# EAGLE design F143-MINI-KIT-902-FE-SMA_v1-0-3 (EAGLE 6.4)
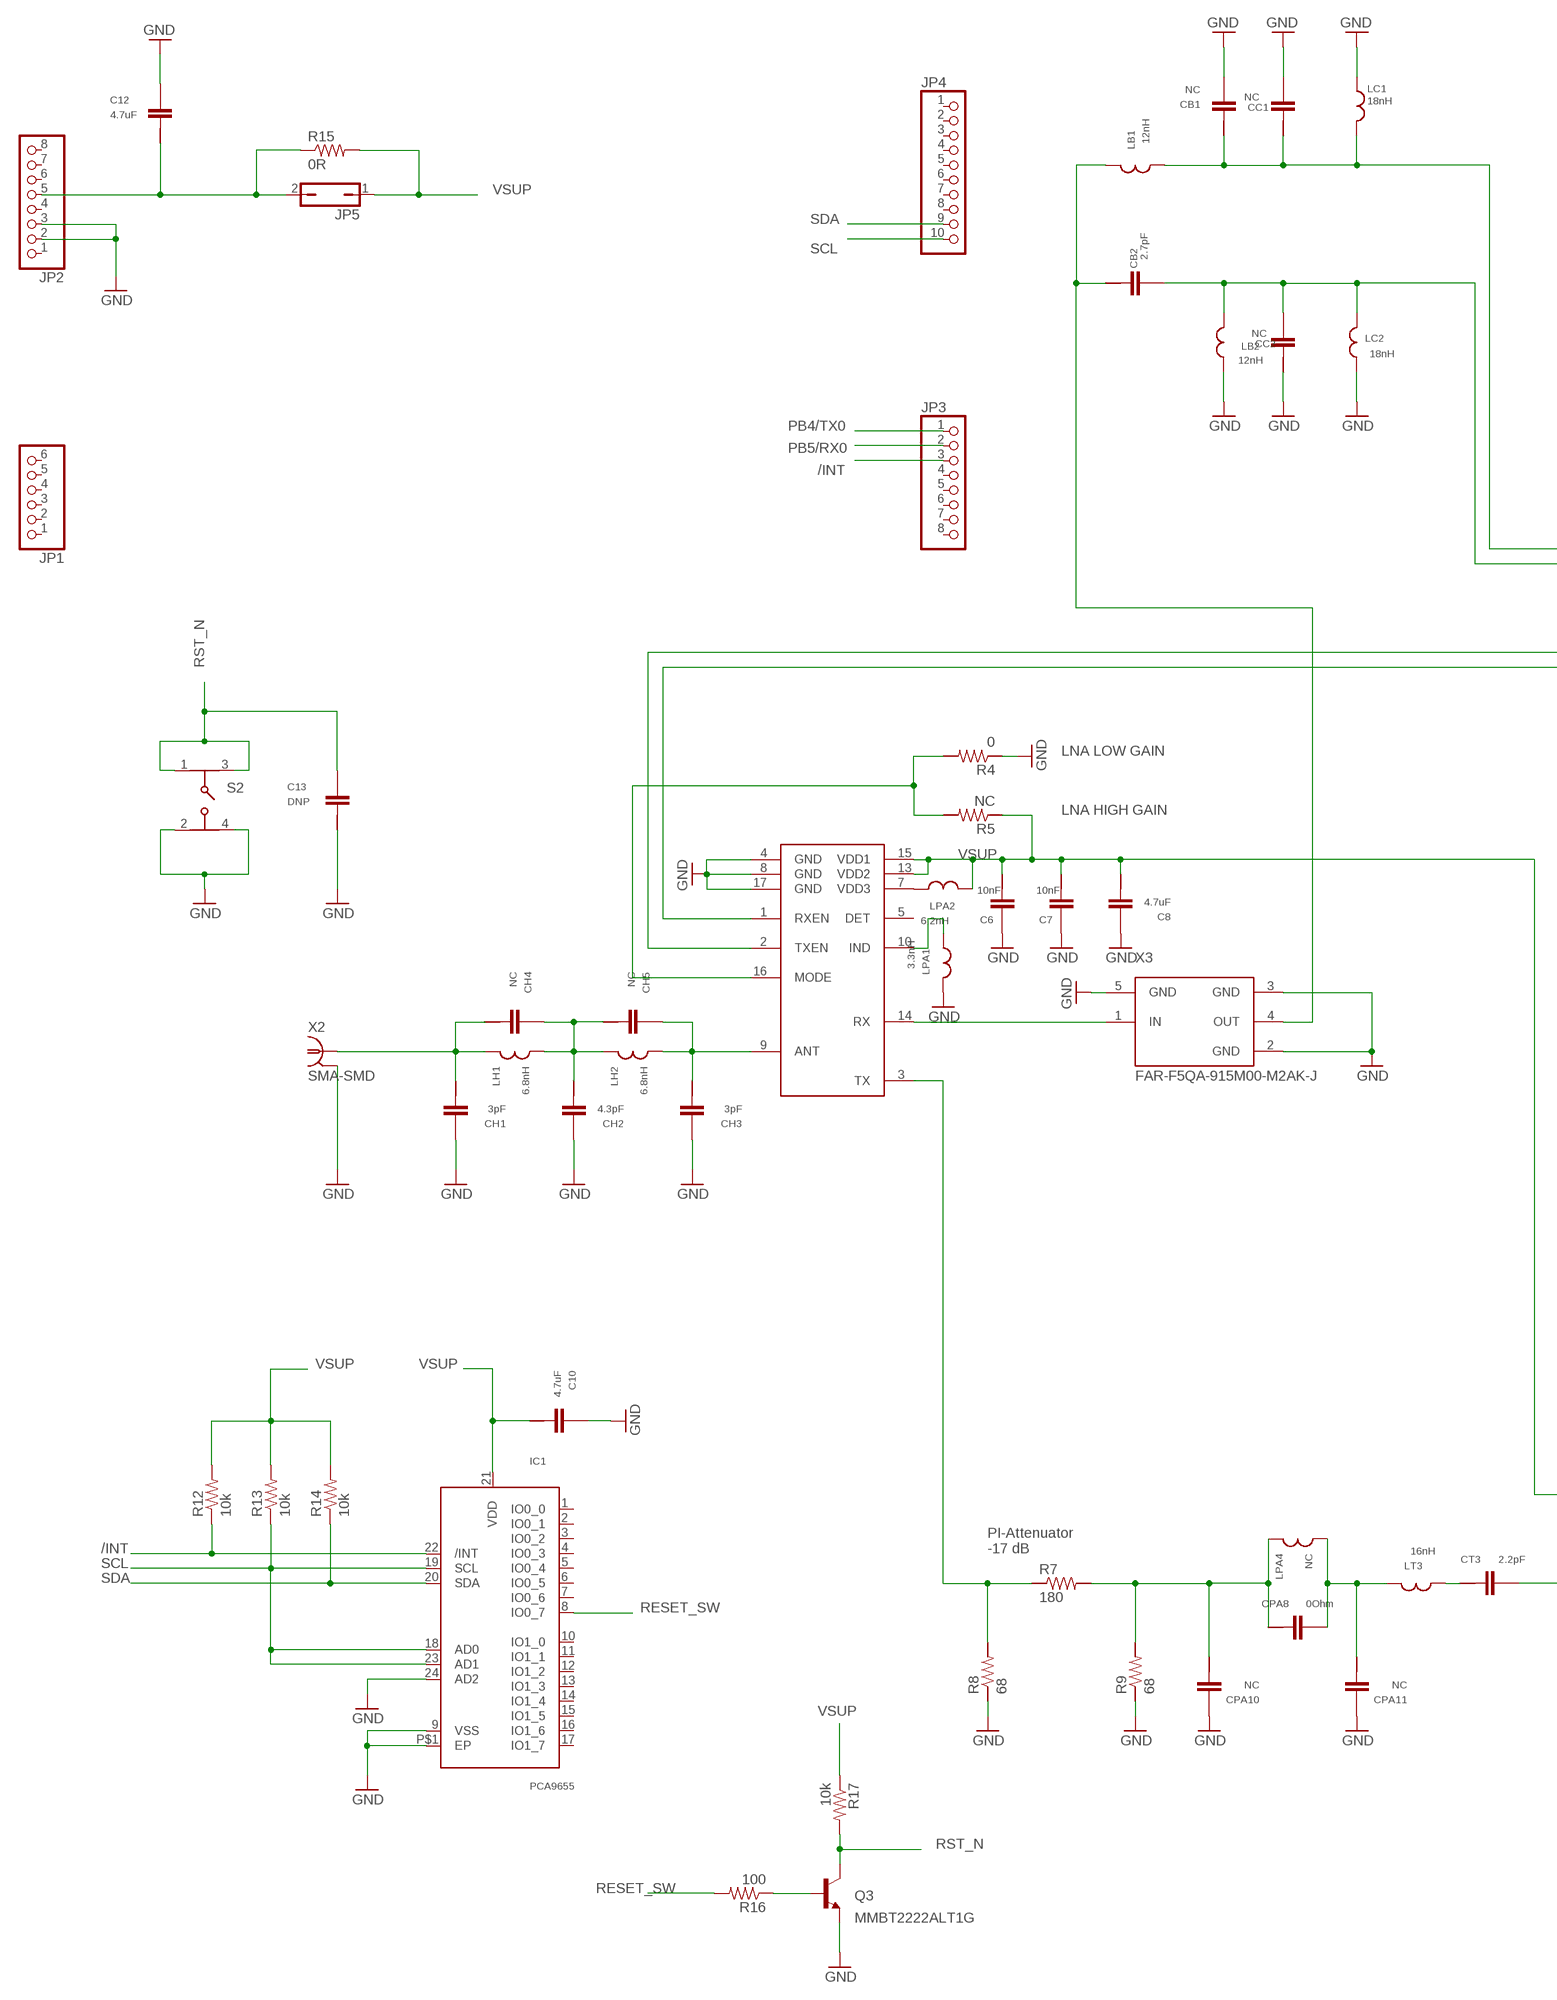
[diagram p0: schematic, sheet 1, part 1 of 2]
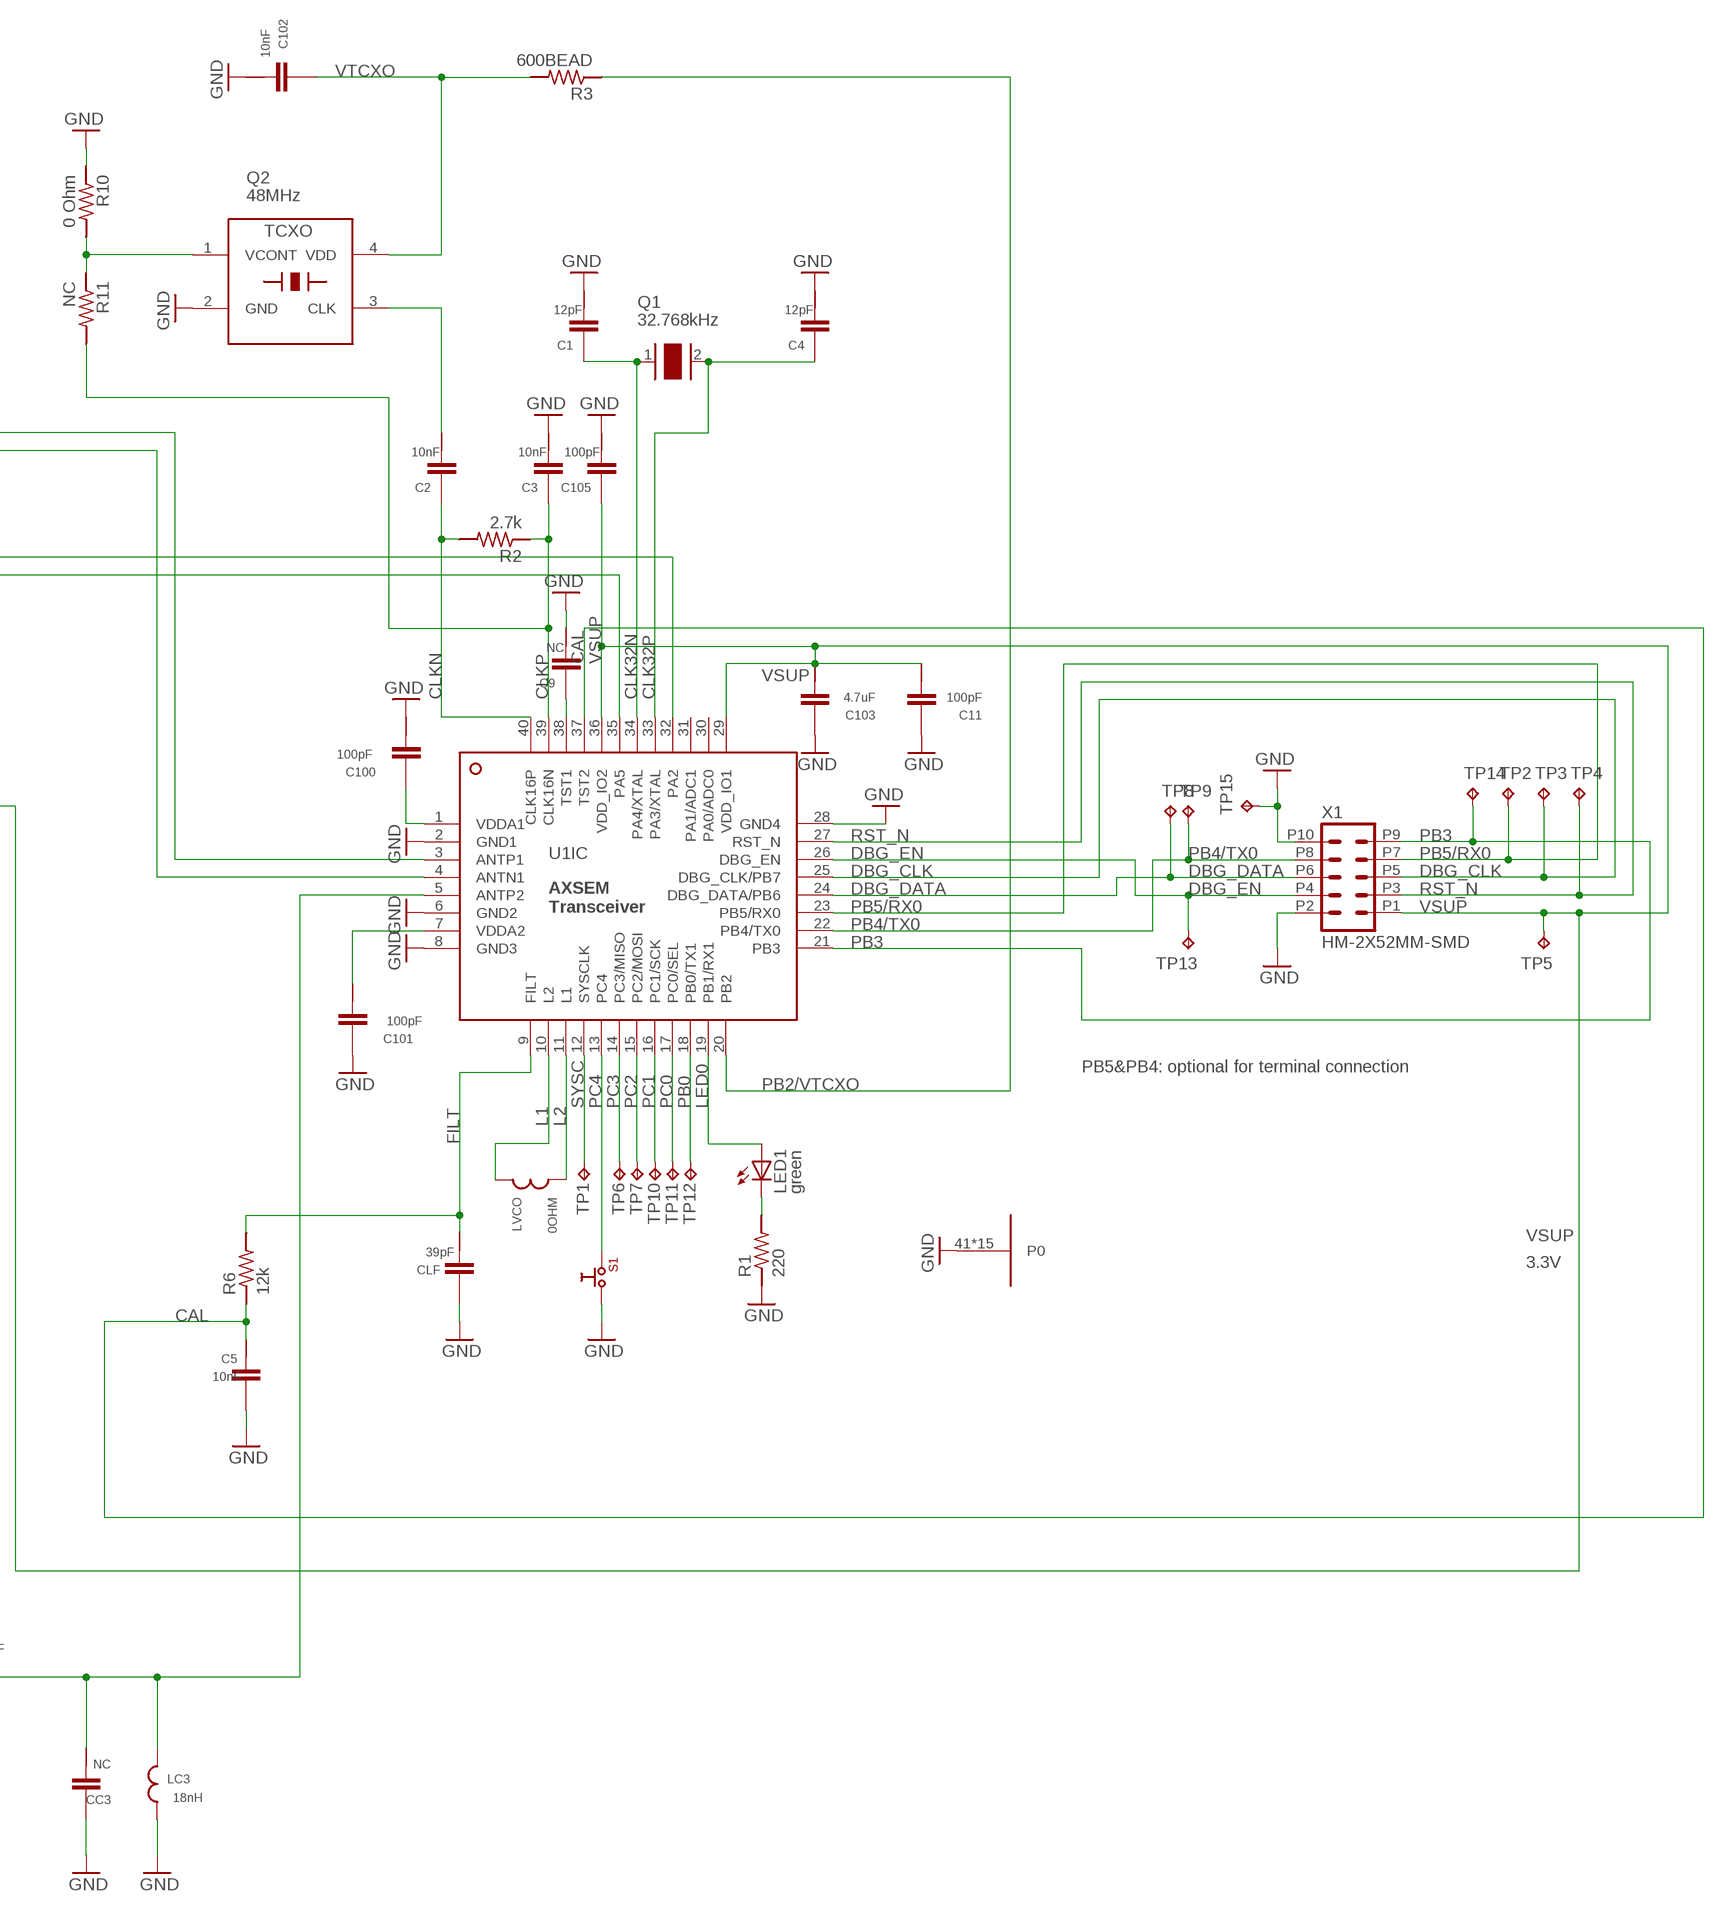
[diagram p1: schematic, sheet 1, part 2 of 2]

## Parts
C1  12pF  C0402  [C0402]
C2  10nF  C0402  [C0402]
C3  10nF  C0402  [C0402]
C4  12pF  C0402  [C0402]
C5  10nF  C0402  [C0402]
C6  10nF  C0402  [C0402]
C7  10nF  C0402  [C0402]
C8  4.7uF  C0603  [C0603]
C9  NC  C0402  [C0402]
C10  4.7uF  C0603  [C0603]
C11  100pF  C0402  [C0402]
C12  4.7uF  C0603  [C0603]
C13  DNP  C0603  [C0603]
C100  100pF  C0402  [C0402]
C101  100pF  C0402  [C0402]
C102  10nF  C0402  [C0402]
C103  4.7uF  C0603  [C0603]
C105  100pF  C0402  [C0402]
CB1  NC  C0402  [C0402]
CB2  2.7pF  C0402  [C0402]
CC1  NC  C0402  [C0402]
CC2  NC  C0402  [C0402]
CC3  NC  C0402  [C0402]
CH1  3pF  C0402  [C0402]
CH2  4.3pF  C0402  [C0402]
CH3  3pF  C0402  [C0402]
CH4  NC  C0402  [C0402]
CH5  NC  C0402  [C0402]
CLF  39pF  C0402  [C0402]
CPA8  0Ohm  C0402  [C0402]
CPA10  NC  C0402  [C0402]
CPA11  NC  C0402  [C0402]
CT3  2.2pF  C0402  [C0402]
IC1  PCA9655  [QFN24]
JP1  PINHD-1X6TH  [1X06-TH]
JP2  PINHD-1X8TH  [1X08-TH]
JP3  PINHD-1X8TH  [1X08-TH]
JP4  PINHD-1X10_ARD  [1X10]
JP5  JP1Q  [JP1]
LB1  12nH  L0402WW  [L0402WW]
LB2  12nH  L0402WW  [L0402WW]
LC1  18nH  L0402WW  [L0402WW]
LC2  18nH  L0402WW  [L0402WW]
LC3  18nH  L0402WW  [L0402WW]
LED1  green  LED0603  [LED0603]
LH1  6.8nH  L0402WW  [L0402WW]
LH2  6.8nH  L0402WW  [L0402WW]
LPA1  3.3nH  L0402WW  [L0402WW]
LPA2  6.2nH  L0402WW  [L0402WW]
LPA4  NC  L0402WW  [L0402WW]
LT3  16nH  L0402WW  [L0402WW]
LVCO  0OHM  L0402WW  [L0402WW]
Q1  32.768kHz  XTAL-2PINTF20  [TF20]
Q2  48MHz  TCXO  [X2016]
Q3  MMBT2222ALT1G  BC817-16LT1SMD  [SOT23-BEC]
R1  220  R0402  [R0402]
R2  2.7k  R0402  [R0402]
R3  600BEAD  R0402  [R0402]
R4  0  R0402  [R0402]
R5  NC  R0402  [R0402]
R6  12k  R0402  [R0402]
R7  180  R0402  [R0402]
R8  68  R0402  [R0402]
R9  68  R0402  [R0402]
R10  0 Ohm  R0402  [R0402]
R11  NC  R0402  [R0402]
R12  10k  R-US_R0603  [R0603]
R13  10k  R-US_R0603  [R0603]
R14  10k  R-US_R0603  [R0603]
R15  0R  R-US_R0603  [R0603]
R16  100  R-US_R0603  [R0603]
R17  10k  R-US_R0603  [R0603]
S1  TASTER4-PAD-SMD-SMALL  [TASTER_SMALL_SMD_4PAD]
S2  430152043826  [430152043826]
TP1  TP03  [PIN-03]
TP2  TPTP10R  [TP10R]
TP3  TPTP10R  [TP10R]
TP4  TPTP10R  [TP10R]
TP5  TPTP10R  [TP10R]
TP6  TP03  [PIN-03]
TP7  TP03  [PIN-03]
TP8  TPTP10R  [TP10R]
TP9  TPTP10R  [TP10R]
TP10  TP03  [PIN-03]
TP11  TP03  [PIN-03]
TP12  TP03  [PIN-03]
TP13  TPTP10R  [TP10R]
TP14  TPTP10R  [TP10R]
TP15  TPTP10R  [TP10R]
U1  AXSEMTRANSCEIVERN  [QFN40]
U$2  RFX1010  [QFN16_TH]
X1  HM-2X52MM-SMD  [HM-2MM-2X5-SMD]
X2  SMA-SMD  [SMA-SMD]
X3  FAR-F5QA-915M00-M2AK-J  WFC30A0915FE  [SAW_1.4X1.1X0.5]

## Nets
/INT: IC1.22(/INT) JP3.3 R12.1
ANT1: CB1.1 CC1.1 LB1.1 LC1.2 U1.3(IC:ANTP1)
ANT2: CB2.2 CC2.2 LB2.2 LC2.2 U1.4(IC:ANTN1)
ANT3: CC3.1 CT3.2 LC3.2 U1.5(IC:ANTP2)
APE_PA: U1.32(IC:PA2) U$2.2(TXEN)
APEN_PA: U1.35(IC:PA5) U$2.1(RXEN)
CAL: C5.1 R6.3 U1.37(IC:TST2)
CLK: C2.1 Q2.3(CLK)
CLK32N: C1.2 Q1.1 U1.34(IC:PA4/XTAL)
CLK32P: C4.2 Q1.2 U1.33(IC:PA3/XTAL)
CLKN: C2.2 R2.4 U1.40(IC:CLK16P)
CLKP: C3.2 R2.3 R11.4 U1.39(IC:CLK16N)
DBG_CLK: TP3.TP U1.25(IC:DBG_CLK/PB7) X1.P5
DBG_DATA: TP8.TP U1.24(IC:DBG_DATA/PB6) X1.P6
DBG_EN: TP13.TP U1.26(IC:DBG_EN) X1.P4
FILT: CLF.1 R6.4 U1.9(IC:FILT)
FPA1: CT3.1 LT3.1
GND: C1.1 C3.1 C4.1 C5.2 C6.2 C7.2 C8.2 C9.1 C10.2 C11.2 C12.2 C13.1 C100.1 C101.2 C102.1 C103.2 C105.1 CB1.2 CC1.2 CC2.1 CC3.2 CH1.2 CH2.2 CH3.2 CLF.2 CPA10.2 CPA11.2 IC1.9(VSS) IC1.24(AD2) IC1.P$1(EP) JP2.2 JP2.3 LB2.1 LC1.1 LC2.1 LC3.1 LPA1.2 Q2.2(GND) Q3.E R1.3 R4.3 R8.3 R9.3 R10.3 S1.P3 S2.2 S2.4 TP15.TP U1.2(IC:GND1) U1.6(IC:GND2) U1.8(IC:GND3) U1.28(IC:GND4) U1.41(GP:P0) U1.42(GP:P0) U1.43(GP:P0) U1.44(GP:P0) U1.45(GP:P0) U1.46(GP:P0) U1.47(GP:P0) U1.48(GP:P0) U1.49(GP:P0) U1.50(GP:P0) U1.51(GP:P0) U1.52(GP:P0) U1.53(GP:P0) U1.54(GP:P0) U1.55(GP:P0) U$2.4(GND) U$2.8(GND) U$2.17(GND) X1.P2 X1.P10 X2.2@1(GND) X3.2(GND) X3.3(GND) X3.5(GND)
L1: LVCO.2 U1.10(IC:L2)
L2: LVCO.1 U1.11(IC:L1)
LED0: LED1.A U1.19(IC:PB1/RX1)
N$1: U$2.14(RX) X3.1(IN)
N$2: LED1.C R1.4
N$3: CH3.1 CH5.2 LH2.2 U$2.9(ANT)
N$4: CH2.1 CH4.2 CH5.1 LH1.2 LH2.1
N$5: CH1.1 CH4.1 LH1.1 X2.1
N$6: R4.4 R5.4 U$2.16(MODE)
N$7: C12.1 JP2.5 JP5.2 R15.1
N$8: LPA1.1 U$2.10(IND)
N$9: LPA2.1 U$2.7(VDD3)
N$10: Q2.1(VCONT) R10.4 R11.3
N$11: C9.2 U1.38(IC:TST1)
N$12: CPA8.1 CPA10.1 LPA4.1 R7.4 R9.4
N$14: R7.3 R8.4 U$2.3(TX)
N$15: Q3.B R16.1
N$17: CPA8.2 CPA11.1 LPA4.2 LT3.2
N$23: CB2.1 LB1.2 X3.4(OUT)
PB0: TP12.P$1(TP) U1.18(IC:PB0/TX1)
PB2/VTCXO: R3.3 U1.20(IC:PB2)
PB3: TP14.TP U1.21(IC:PB3) X1.P9
PB4/TX0: JP3.1 TP9.TP U1.22(IC:PB4/TX0) X1.P8
PB5/RX0: JP3.2 TP2.TP U1.23(IC:PB5/RX0) X1.P7
PC0: TP11.P$1(TP) U1.17(IC:PC0/SEL)
PC1: TP10.P$1(TP) U1.16(IC:PC1/SCK)
PC2: TP7.P$1(TP) U1.15(IC:PC2/MOSI)
PC3: TP6.P$1(TP) U1.14(IC:PC3/MISO)
PC4: S1.P1 U1.13(IC:PC4)
RESET_SW: IC1.8(IO0_7) R16.2
RST_N: C13.2 Q3.C R17.2 S2.1 S2.3 TP4.TP U1.27(IC:RST_N) X1.P3
SCL: IC1.18(AD0) IC1.19(SCL) IC1.23(AD1) JP4.10 R13.1
SDA: IC1.20(SDA) JP4.9 R14.1
SYSC: TP1.P$1(TP) U1.12(IC:SYSCLK)
VDDA1: C100.2 U1.1(IC:VDDA1)
VDDA2: C101.1 U1.7(IC:VDDA2)
VSUP: C6.1 C7.1 C8.1 C10.1 C11.1 C103.1 C105.2 IC1.21(VDD) JP5.1 LPA2.2 R5.3 R12.2 R13.2 R14.2 R15.2 R17.1 TP5.TP U1.29(IC:VDD_IO1) U1.36(IC:VDD_IO2) U$2.13(VDD2) U$2.15(VDD1) X1.P1
VTCXO: C102.2 Q2.4(VDD) R3.4
Unconnected: IC1.1(IO0_0) IC1.2(IO0_1) IC1.3(IO0_2) IC1.4(IO0_3) IC1.5(IO0_4) IC1.6(IO0_5) IC1.7(IO0_6) IC1.10(IO1_0) IC1.11(IO1_1) IC1.12(IO1_2) IC1.13(IO1_3) IC1.14(IO1_4) IC1.15(IO1_5) IC1.16(IO1_6) IC1.17(IO1_7) JP1.1 JP1.2 JP1.3 JP1.4 JP1.5 JP1.6 JP2.1 JP2.4 JP2.6 JP2.7 JP2.8 JP3.4 JP3.5 JP3.6 JP3.7 JP3.8 JP4.1 JP4.2 JP4.3 JP4.4 JP4.5 JP4.6 JP4.7 JP4.8 U1.30(IC:PA0/ADC0) U1.31(IC:PA1/ADC1) U$2.5(DET)

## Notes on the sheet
- LNA LOW GAIN
- LNA HIGH GAIN
- PB5&PB4: optional for terminal connection
- 3.3V
- PI-Attenuator
  -17 dB

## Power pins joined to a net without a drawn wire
GND: X2.2@2(GND) X2.2@3(GND) X2.2@4(GND) X2.2@5(GND) X2.2@6(GND)

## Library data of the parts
C1-C7 C9 C11 C100 C101 C105 CB1 CB2 CC1-CC3 CH1-CH5 CLF CPA8 CPA10 CPA11 CT3 = axsem_passives_v1-4:C
C8 C10 C12 C13 C102 C103 = axsem_passives_v1-5:C
IC1 = IoT small BB_SigFox chips:PCA9655
JP1 = SmartPrj:PINHD-1X6: PIN HEADER
JP2 JP3 = SmartPrj:PINHD-1X8: PIN HEADER
JP4 = SmartPrj:PINHD-1X10_ARD: PIN HEADER
JP5 = jumper:JP1Q: JUMPER
LB1 LB2 LC1-LC3 LH1 LH2 LPA1 LPA2 LPA4 LT3 LVCO = axsem_passives_v1-7:L
LED1 = axsem_passives_v1-4:LED
Q1 = axsem_osc_v1-2:XTAL-2PIN
Q2 = axsem_osc_v1-3:TCXO
Q3 = transistor-npn:BC817*: NPN Transistor
R1-R11 = axsem_passives_v1-4:R
R12-R17 = resistor:R-US_: RESISTOR, American symbol
S1 = axsem_switches_v1.2:TASTER: AXSEM tasters
S2 = EAGLE-TACT_SWITCHES-rev17a:430152043826: 6x6 mm SMD WS-TASV Details see: http://katalog.we-online.de/em/datasheet/4301x2xxx8x6.pdf 2015 (C) Würth Elektronik
TP1 TP6 TP7 TP10-TP12 = axsem_testpad_v1-0:TP: Test pad
TP2-TP5 TP8 TP9 TP13-TP15 = testpad:TP: Test pad
U1 = axsem_v4-25:AXSEMTRANSCEIVER: RF-MICRO
U$2 = axsem_rf_v1-3:RFX1010
X1 = axsem_connectors_v1-5:HM-2X5
X2 = axsem_connectors_v1-5:SMA-SMD: SMA 50 Ohm Straight Jack Receptacle - Surface Mount www.johnsoncomponents.com Source: http://catalog.digikey.com .. 142-0711-201, 205, 202, 206.pdf
X3 = axsem_rf_v1-3:WFC30A0915FE

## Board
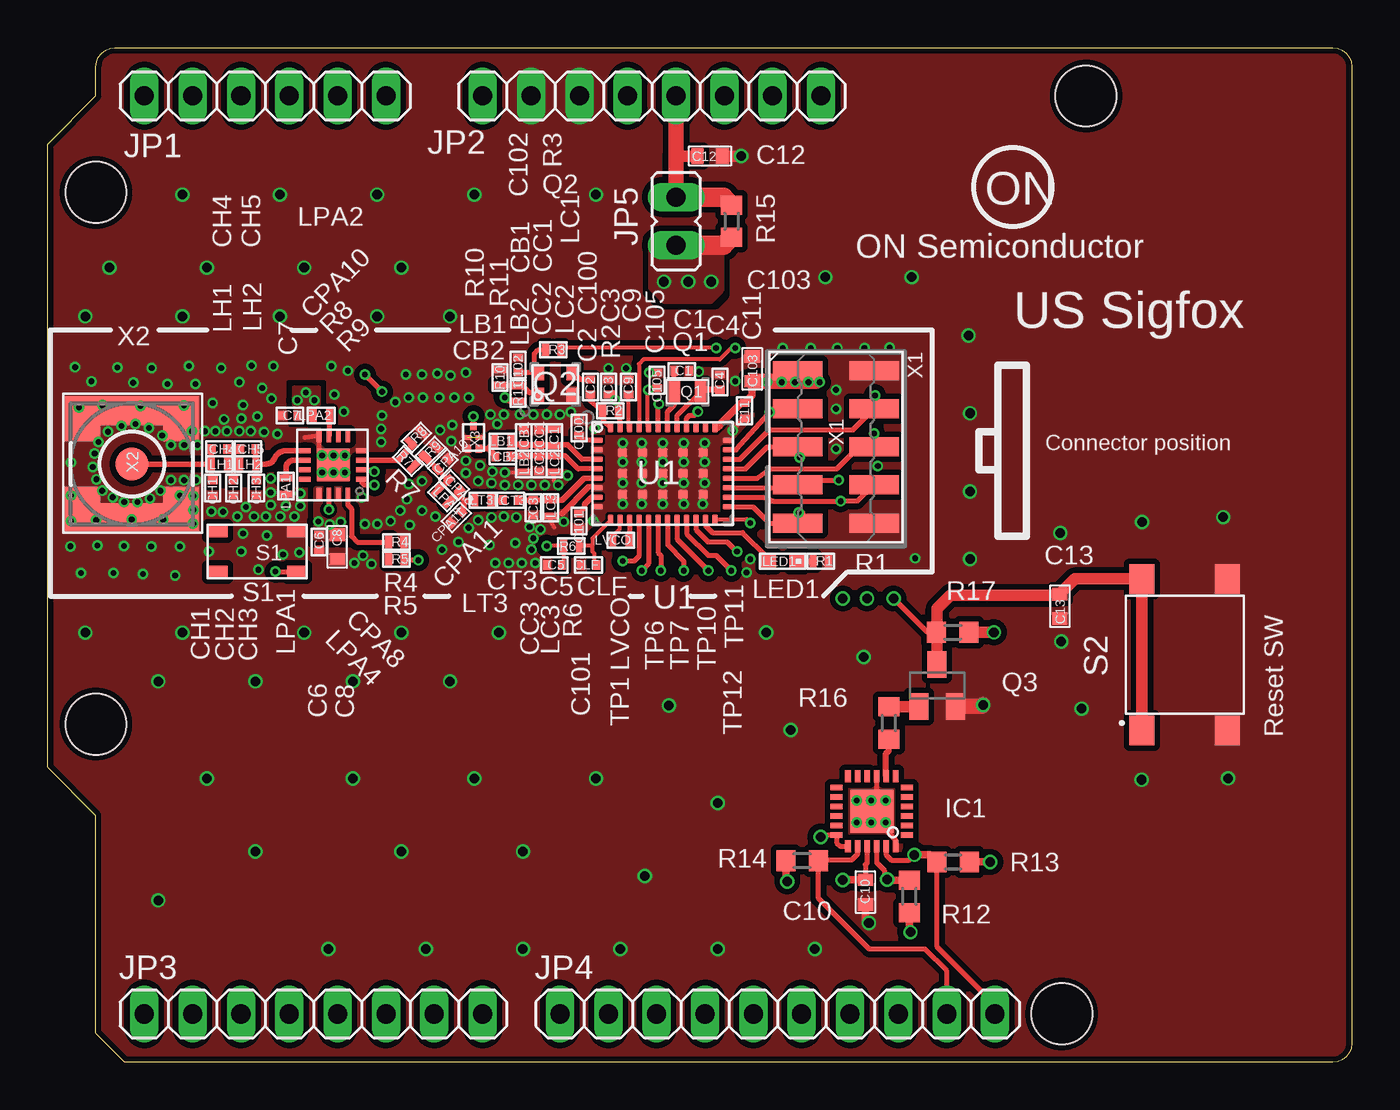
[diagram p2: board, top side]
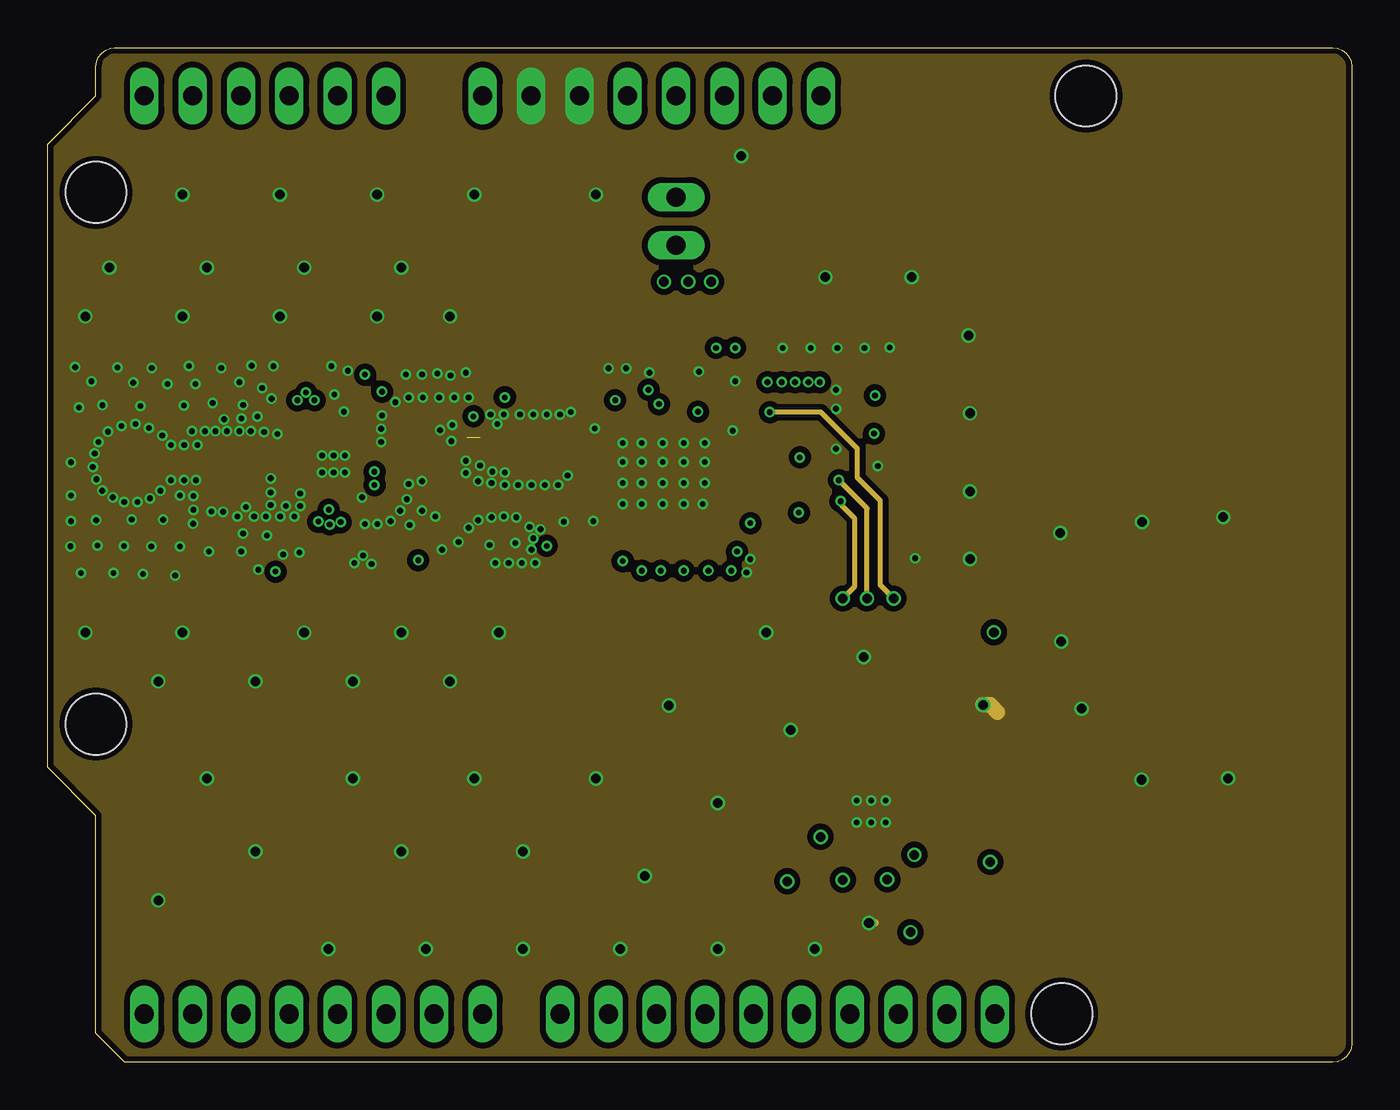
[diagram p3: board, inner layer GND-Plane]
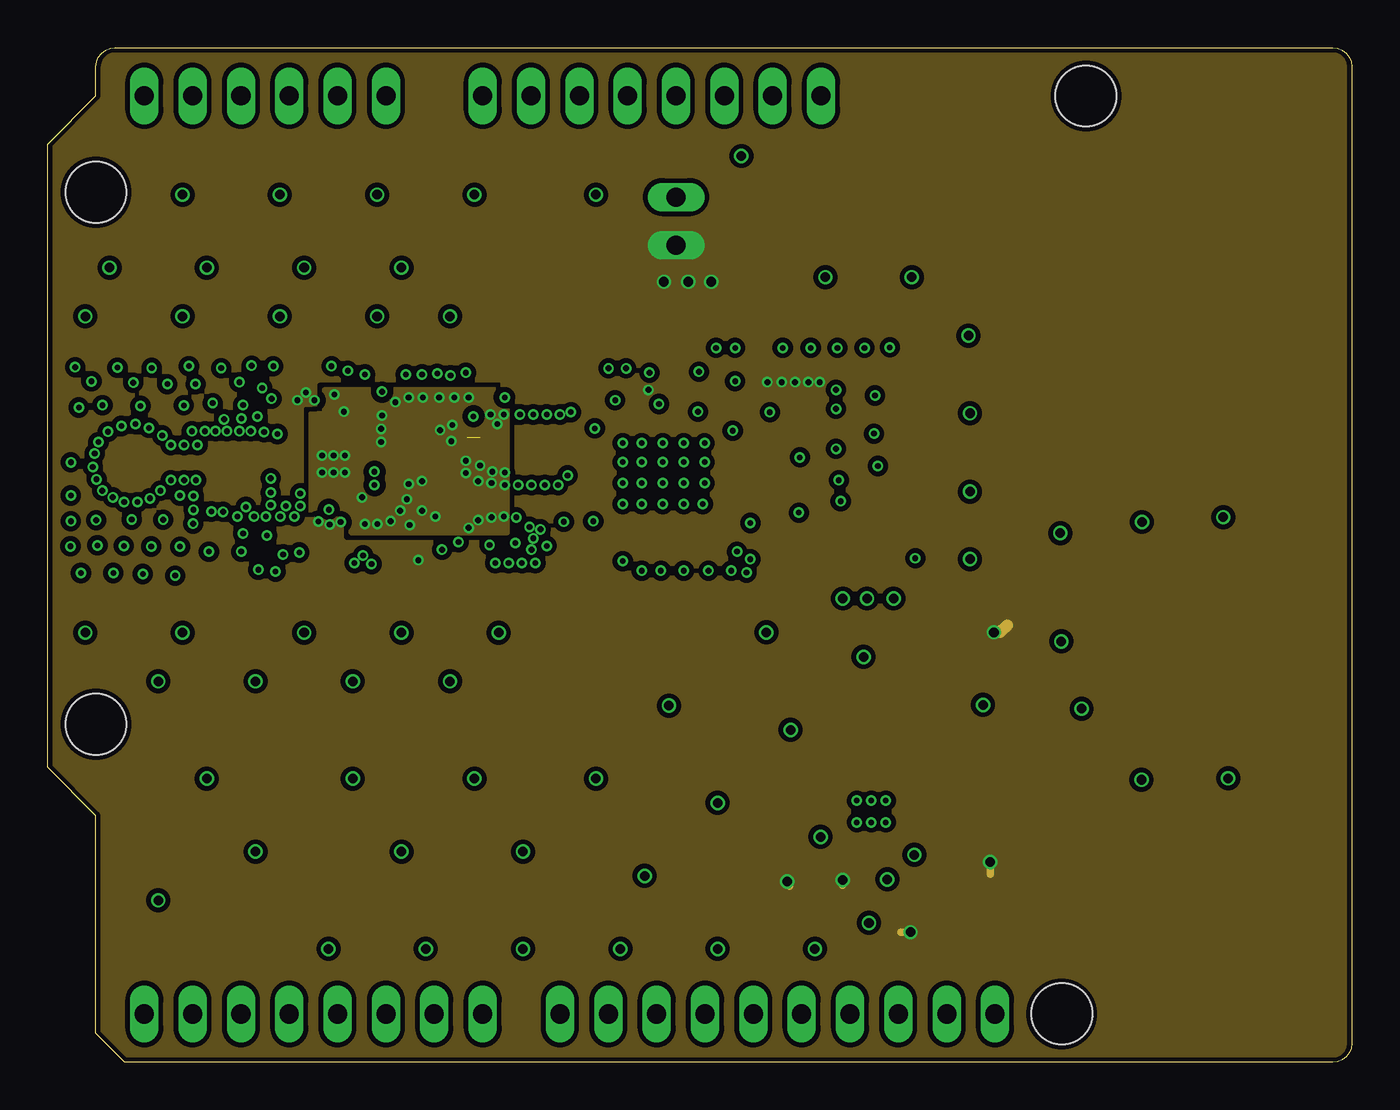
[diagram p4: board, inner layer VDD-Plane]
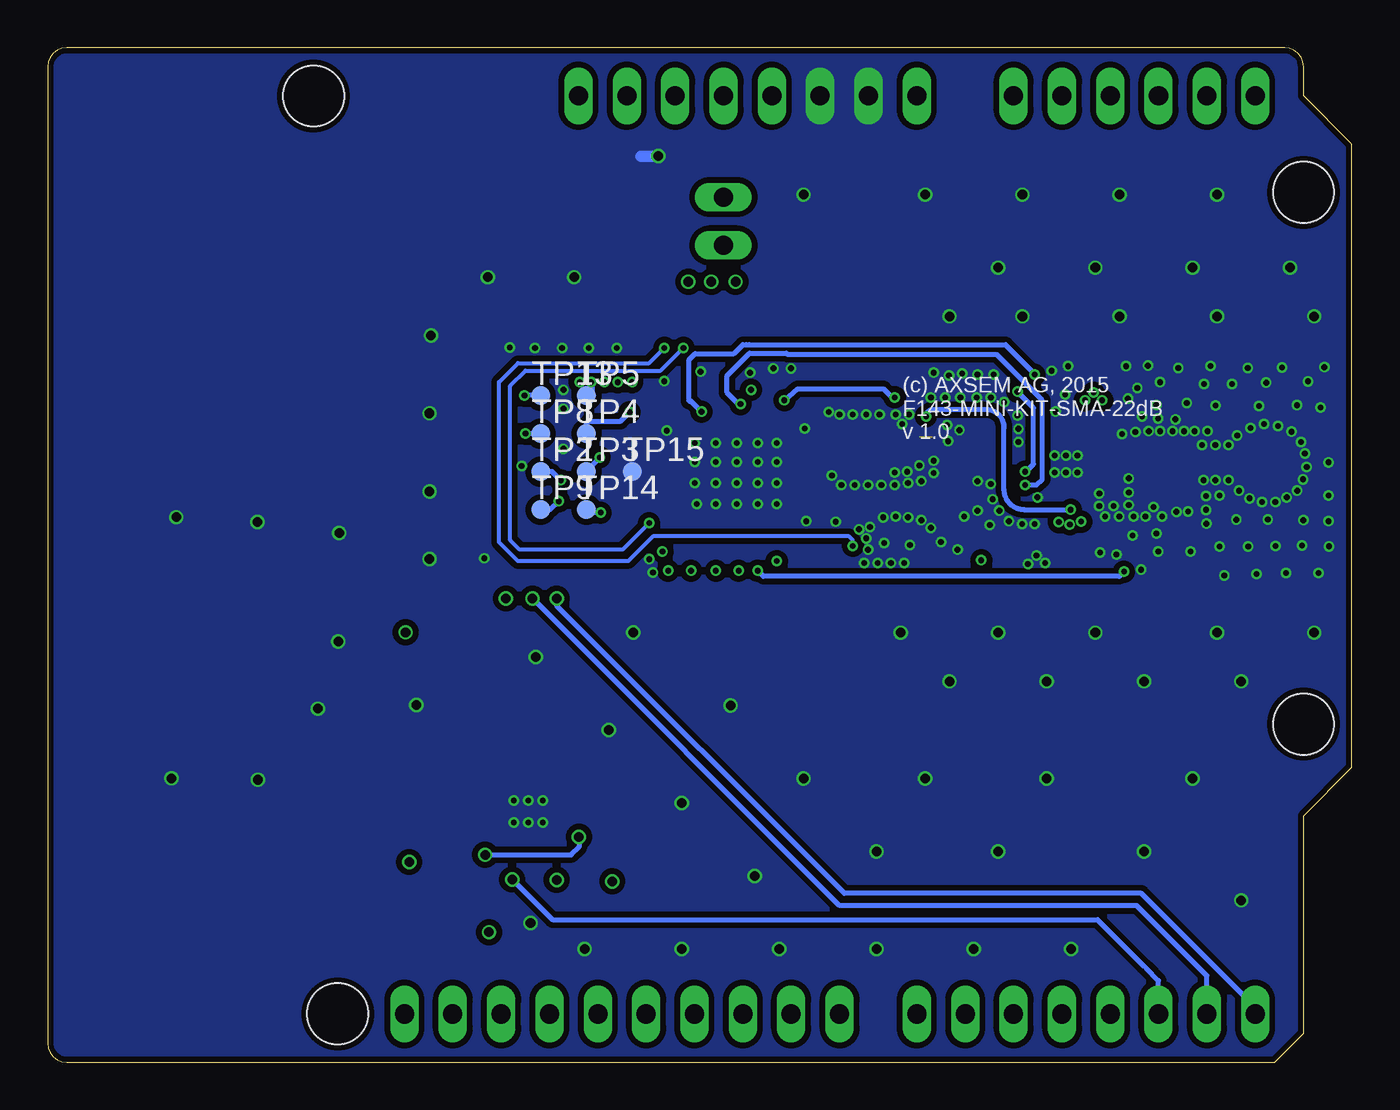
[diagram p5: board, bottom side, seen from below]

Size 68.53 x 53.3 mm. Coordinates in mm from the lower left corner, seen from the top.
Outline: 67.54,0 4.06,0 2.54,1.52 2.54,12.95 0,15.49 0,48.22 2.54,50.76 2.54,52.31 2.58,52.56 2.67,52.79 2.84,53 3.05,53.17 3.28,53.26 3.53,53.3 67.54,53.3 67.79,53.26 68.03,53.17 68.24,53 68.41,52.79 68.49,52.56 68.53,52.31 68.53,1.02 68.49,0.74 68.41,0.51 68.24,0.3 68.03,0.15 67.79,0.04 67.54,0
Copper layers (1+2*3+16): Top 0.018mm / dielectric 0.36mm / GND-Plane 0.035mm / dielectric 0.71mm / VDD-Plane 0.035mm / dielectric 0.36mm / Bottom 0.018mm
Design rules "Multi-CB_4L_125µm-Tracks_OL35µm-IL35µm *": minimum track width 0.125mm, minimum drill 0.2mm, track to track 0.125mm, track to pad 0.125mm, pad to pad 0.125mm, via to via 0.125mm, smd to smd 0mil, copper to edge 0.2mm, drill to drill 0.2mm, minimum pad ring 0.125mm, minimum via ring 0.125mm, stop-mask expansion 2mil, vias tented up to drill 0.45mm, thermal gap 0.2mm
Holes 3.2 mm at 2.54,17.76 2.54,45.7 54.56,50.76 53.29,2.55

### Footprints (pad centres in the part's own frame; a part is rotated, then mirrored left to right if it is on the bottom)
C0402 = smd 0.4 x 0.5: 1 -0.4,0; 2 0.4,0
C0603 = smd 0.65 x 0.8: 1 -0.65,0; 2 0.65,0
QFN24 = smd 0.63 x 0.3: 1 -1.85,1.25; 2 -1.85,0.75; 3 -1.85,0.25; 4 -1.85,-0.25; 5 -1.85,-0.75; 6 -1.85,-1.25; 13 1.85,-1.25; 14 1.85,-0.75; 15 1.85,-0.25; 16 1.85,0.25; 17 1.85,0.75; 18 1.85,1.25 | smd 0.3 x 0.63: 7 -1.25,-1.85; 8 -0.75,-1.85; 9 -0.25,-1.85; 10 0.25,-1.85; 11 0.75,-1.85; 12 1.25,-1.85; 19 1.25,1.85; 20 0.75,1.85; 21 0.25,1.85; 22 -0.25,1.85; 23 -0.75,1.85; 24 -1.25,1.85 | smd 2.26 x 2.26: P$1 0,0
1X06-TH = drill 1 pad 1.422 long: 1 -6.35,0; 2 -3.81,0; 3 -1.27,0; 4 1.27,0; 5 3.81,0; 6 6.35,0
1X08-TH = drill 1 pad 1.422 long: 1 -8.89,0; 2 -6.35,0; 3 -3.81,0; 4 -1.27,0; 5 1.27,0; 6 3.81,0; 7 6.35,0; 8 8.89,0
1X10 = drill 1 pad 1.422 long: 1 -11.43,0; 2 -8.89,0; 3 -6.35,0; 4 -3.81,0; 5 -1.27,0; 6 1.27,0; 7 3.81,0; 8 6.35,0; 9 8.89,0; 10 11.43,0
JP1 = drill 1 long: 1 0,-1.27; 2 0,1.27
L0402WW = smd 0.35 x 0.65: 1 -0.425,0; 2 0.425,0
LED0603 = smd 0.8 x 0.8: A -0.75,0; C 0.75,0
TF20 = smd 0.6 x 1.1: 1 -0.7,0; 2 0.7,0
X2016 = smd 0.6 x 0.8: 1 -0.9,-0.6; 2 0.9,-0.6; 3 0.9,0.6; 4 -0.9,0.6
SOT23-BEC = smd 1 x 1.4: B -0.95,-1.1; C 0,1.1; E 0.95,-1.1
R0402 = smd 0.36 x 0.66: 3 -0.41,0; 4 0.41,0
R0603 = smd 1 x 1.1: 1 -0.85,0; 2 0.85,0
TASTER_SMALL_SMD_4PAD = smd 1.05 x 0.65: P1 -2.075,1.075; P2 2.075,1.075; P3 -2.075,-1.075; P4 2.075,-1.075
430152043826 = smd 1.55 x 1.3: 1 -3.975,2.25; 2 -3.975,-2.25; 3 3.975,2.25; 4 3.975,-2.25
PIN-03 = drill 0.3: P$1 0,0
TP10R = smd 1 x 1: TP 0,0
QFN40 = smd 0.5 x 0.3: 1 -3.4,1.75; 2 -3.4,1.25; 3 -3.4,0.75; 4 -3.4,0.25; 5 -3.4,-0.25; 6 -3.4,-0.75; 7 -3.4,-1.25; 8 -3.4,-1.75; 21 3.4,-1.75; 22 3.4,-1.25; 23 3.4,-0.75; 24 3.4,-0.25; 25 3.4,0.25; 26 3.4,0.75; 27 3.4,1.25; 28 3.4,1.75 | smd 0.3 x 0.5: 9 -2.75,-2.4; 10 -2.25,-2.4; 11 -1.75,-2.4; 12 -1.25,-2.4; 13 -0.75,-2.4; 14 -0.25,-2.4; 15 0.25,-2.4; 16 0.75,-2.4; 17 1.25,-2.4; 18 1.75,-2.4; 19 2.25,-2.4; 20 2.75,-2.4; 29 2.75,2.4; 30 2.25,2.4; 31 1.75,2.4; 32 1.25,2.4; 33 0.75,2.4; 34 0.25,2.4; 35 -0.25,2.4; 36 -0.75,2.4; 37 -1.25,2.4; 38 -1.75,2.4; 39 -2.25,2.4; 40 -2.75,2.4 | smd 0.5 x 0.5: 41 -2.12,1.1; 42 -2.12,0; 43 -2.12,-1.1; 44 -1.06,1.1; 45 -1.06,0; 46 -1.06,-1.1; 47 0,1.1; 48 0,0; 49 0,-1.1; 50 1.06,-1.1; 51 1.06,0; 52 1.06,1.1; 53 2.12,-1.1; 54 2.12,0; 55 2.12,1.1
QFN16_TH = smd 0.6 x 0.25: 1 -1,0.5; 2 -1,0; 3 -1,-0.5; 4 -1,-1; 9 2,-1; 10 2,-0.5; 11 2,0; 12 2,0.5 | smd 0.25 x 0.6: 5 -0.25,-1.75; 6 0.25,-1.75; 7 0.75,-1.75; 8 1.25,-1.75; 13 1.25,1.25; 14 0.75,1.25; 15 0.25,1.25; 16 -0.25,1.25 | smd 1.7 x 1.7: 17 0.5,-0.25
HM-2MM-2X5-SMD = smd 1 x 2.6: P1 -4,-2; P2 -4,2; P3 -2,-2; P4 -2,2; P5 0,-2; P6 0,2; P7 2,-2; P8 2,2; P9 4,-2; P10 4,2
SMA-SMD = smd 1.73 x 1.73: 1 0,0 | smd 2.35 x 1.9: 2@1 -2.375,2.6; 2@2 -2.375,-2.6; 2@3 2.375,-2.6; 2@4 2.375,2.6 | smd 1.5 x 3.4: 2@5 -2.8,0; 2@6 2.8,0
SAW_1.4X1.1X0.5 = smd 0.425 x 0.325: 1 -0.588,0; 3 0.588,-0.287; 4 0.588,0.287 | smd 0.25 x 0.425: 2 0,-0.338; 5 0,0.338

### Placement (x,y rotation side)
C1  33.32,36.33 180 top
C2  28.52,35.48 270 top
C3  29.47,35.48 270 top
C4  35.32,35.73 270 top
C5  26.62,26.13 180 top
C6  14.27,27.33 270 top
C7  12.72,33.98 180 top
C8  15.22,27.08 270 top
C9  30.52,35.48 270 top
C10  42.97,8.94 270 top
C11  36.62,34.23 270 top
C12  34.8,47.61 0 top
C13  53.19,23.96 90 top
C100  27.92,33.33 270 top
C101  27.92,28.43 270 top
C102  24.72,36.63 270 top
C103  37.02,36.43 90 top
C105  32.02,35.83 270 top
CB1  25.02,32.83 90 top
CB2  23.92,31.83 0 top
CC1  25.82,32.83 90 top
CC2  25.82,31.43 90 top
CC3  25.52,29.13 270 top
CH1  8.67,30.18 270 top
CH2  9.77,30.18 270 top
CH3  10.97,30.18 270 top
CH4  9.02,32.23 0 top
CH5  10.52,32.23 0 top
CLF  28.42,26.13 180 top
CPA8  21.37,30.33 315 top
CPA10  20.77,31.43 45 top
CPA11  21.47,28.63 225 top
CT3  24.32,29.53 0 top
IC1  43.31,13.19 180 top
JP1  11.43,50.76 0 top
JP2  31.75,50.76 0 top
JP3  13.97,2.54 0 top
JP4  38.35,2.54 0 top
JP5  33.02,44.18 0 top
LB1  23.92,32.63 180 top
LB2  25.02,31.43 90 top
LC1  26.62,32.83 270 top
LC2  26.62,31.43 90 top
LC3  26.42,29.13 90 top
LED1  38.62,26.33 0 top
LH1  9.02,31.43 0 top
LH2  10.52,31.43 0 top
LPA1  12.52,30.28 270 top
LPA2  14.37,33.98 180 top
LPA4  20.77,29.73 315 top
LT3  22.87,29.53 180 top
LVCO  30.12,27.43 180 top
Q1  33.62,35.23 0 top
Q2  26.67,35.63 0 top
Q3  46.74,19.79 0 top
R1  40.62,26.33 180 top
R2  29.57,34.23 180 top
R3  26.57,37.43 180 top
R4  18.32,27.33 180 top
R5  18.32,26.43 180 top
R6  27.52,27.13 0 top
R7  18.92,31.58 315 top
R8  19.37,32.83 225 top
R9  20.12,32.08 225 top
R10  23.77,35.98 270 top
R11  24.72,35.13 270 top
R12  45.28,8.71 270 top
R13  47.58,10.52 0 top
R14  39.65,10.6 180 top
R15  35.94,44.18 270 top
R16  44.2,17.82 270 top
R17  47.56,22.59 180 top
S1  11.02,26.83 180 top
S2  59.74,21.42 90 top
TP1  30.22,26.33 0 top
TP2  42.62,31.03 0 bottom
TP3  40.22,31.03 0 bottom
TP4  40.22,33.03 0 bottom
TP5  40.22,35.03 0 bottom
TP6  32.22,25.83 0 top
TP7  33.42,25.83 0 top
TP8  42.62,33.03 0 bottom
TP9  42.62,29.03 0 bottom
TP10  34.72,25.83 95.6 top
TP11  35.92,25.83 90 top
TP12  36.22,26.83 0 top
TP13  42.62,35.03 0 bottom
TP14  40.22,29.03 0 bottom
TP15  37.82,31.03 0 bottom
U1  32.32,30.93 0 top
U$2  15.52,31.13 180 top
X1  41.42,32.33 270 top
X2  4.42,31.43 90 top
X3  22.37,32.83 270 top

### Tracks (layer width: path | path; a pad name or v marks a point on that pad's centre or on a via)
/INT  (via drill 0.5)
  Top 0.254: 44.17,9.56 v44.12,9.61 43.97,9.76 43.97,10.09 43.56,10.5 IC1.22
  Top 0.406: R12.1 44.17,9.56
  Bottom 0.254: JP3.3 10.16,4.29 10.8,4.93 10.92,5.06 13.36,7.5 42.01,7.5 v44.12,9.61
ANT1
  Top 0.25: U1.3 28.07,31.68 27.32,32.43 | 26.63,32.43 LC1.2
  Top 0.254: 26.66,32.38 LC1.2
  Top 0.3: 27.32,32.43 26.65,32.43 LC1.2 25.85,32.4 CC1.1
  Top 0.305: CC1.1 CB1.1 24.53,32.43 LB1.1
ANT2
  Top 0.25: U1.4 27.87,31.18 27.17,31.88 26.66,31.88
  Top 0.254: 26.66,31.88 LC2.2
  Top 0.305: CB2.2 LB2.2 CC2.2 | LC2.2 CC2.2 | CC2.2
ANT3
  Top 0.3: U1.5 28.17,30.68 27.02,29.53 27.01,29.54 26.81,29.54 | LC3.2 CC3.1 CT3.2
  Top 0.305: 26.81,29.54 LC3.2
APE_PA  (via drill 0.3)
  Top 0.254: U1.32 33.57,33.83 33.72,33.98 33.97,33.98 v34.17,34.18 | U$2.2 17.07,31.13 v17.17,31.03 | v17.57,35.23 v16.67,36.13
  Bottom 0.254: v34.17,34.18 34.72,34.73 34.82,34.73 34.82,36.91 34.51,37.23 32.47,37.23 32,37.7 31.82,37.7 31.67,37.7 18.2,37.7 16.67,36.18 v16.67,36.13 | v17.17,31.03 17.12,31.03 16.72,31.43 16.72,34.38 v17.57,35.23
APEN_PA  (via drill 0.3)
  Top 0.254: U1.35 32.07,34.48 v32.12,34.58 | U$2.1 16.52,30.43 16.62,30.33 v17.17,30.33
  Bottom 0.254: v32.12,34.58 32.22,34.58 32.82,35.18 32.82,36.08 31.65,37.26 29.72,37.26 29.66,37.19 18.69,37.19 16.27,34.78 16.27,30.63 16.57,30.33 v17.17,30.33
CAL  (via drill 0.3)
  Top 0.2: C5.1 27.11,26.13 R6.3 v26.22,27.13 | v36.12,37.53 35.92,37.53 35.32,36.93 31.32,36.93 31.07,36.68 U1.37
  Bottom 0.2: v26.22,27.13 26.22,27.43 26.42,27.63 36.72,27.63 38.02,26.33 43.82,26.33 44.82,27.33 44.82,35.73 43.82,36.73 36.92,36.73 v36.12,37.53
CLK
  Top 0.254: Q2.3 27.72,36.23 27.97,35.88 C2.1
CLK32N
  Top 0.254: C1.2 Q1.1 32.92,34.53 32.57,34.18 U1.34
CLK32P
  Top 0.254: U1.33 33.07,33.98 Q1.2
  Top 0.305: C4.2 34.42,35.33 Q1.2
CLKN
  Top 0.254: U1.40 29.21,33.69 R2.4 28.52,34.73 C2.2
CLKP  (via drill 0.3)
  Top 0.254: U1.39 30.07,34.29 R2.3 29.98,34.72 C3.2 29.72,35.18 v29.82,34.78 | R11.4 24.22,34.73 v24.02,34.93
  Bottom 0.254: v29.82,34.78 29.12,35.38 24.62,35.38 24.17,34.93 v24.02,34.93
DBG_CLK  (via drill 0.3)
  Top 0.254: U1.25 36.67,31.18 37.82,32.33 X1.P5 39.52,32.23 v39.52,31.78 39.52,31.83
  Bottom 0.254: TP3.TP 39.52,31.73 v39.52,31.78
DBG_DATA  (via drill 0.3)
  Top 0.254: U1.24 37.27,30.68 37.97,31.18 41.47,31.18 42.27,31.98 42.27,32.03 42.37,32.13 42.87,32.13 | 42.87,32.13 42.77,32.03 42.37,32.03 | 43.42,32.43 X1.P6 43.37,32.38 43.42,32.43 | 43.42,32.43 v43.42,33.03 43.42,32.68 42.87,32.13
  Bottom 0.254: TP8.TP v43.42,33.03
DBG_EN  (via drill 0.3)
  Top 0.254: U1.26 36.37,31.68 37.92,33.23 42.32,33.23 X1.P4 43.42,35.03 v43.47,35.03
  Bottom 0.254: TP13.TP v43.47,35.03
FILT
  Top 0.2: U1.9 29.57,28.48 28.62,27.53 28.62,27.13 | CLF.1 28.72,26.23 28.72,26.73 28.62,26.83 28.62,27.13 | 28.62,27.13 R6.4
FPA1
  Top 0.3: CT3.1 LT3.1
GND  (via drill 0.3, 0.3 pad 0.3, 0.5)  (1 unrouted)
  Top 0.2: 26.62,28.1 26.42,28.43 LC3.1 | v26.82,30.33 26.62,30.53 LC2.1 | LB2.1 25,30.98 v24.02,30.98 | LC1.1 26.6,33.23 CC1.2 | C11.2 36.12,33.33 v36,33.18
  Top 0.254: 13.52,32.83 14.27,32.93 U$2.8 14.27,31.98 v14.42,31.88 | IC1.9 43.56,13.7 43.31,13.44 IC1.P$1 44.14,12.36 44.14,12.11 44.56,11.68 IC1.24
  Top 0.3: 28.62,30.23 28.42,30.23 27.02,28.83 | v12.52,29.23 12.55,29.33 LPA1.2
  Top 0.406: C10.2 42.97,7.51 v43.16,7.32
  Top 0.61: C12.2 v36.45,47.61
  Top 0.813: Q3.E 49.07,18.69 v49.15,18.78
  GND-Plane 0.406: v43.16,7.32 43.46,7.32
  GND-Plane 0.813: v49.15,18.78 49.53,18.78 49.91,18.4
  Bottom 0.61: v36.45,47.61 37.34,47.61
  other vias: 41.42,35.33 43.62,31.33 36.92,26.43 41.5,37.53 42.92,37.53 44.25,37.55 38.62,37.53 41.42,34.33 28.75,33.3 41.42,32.23 30.22,32.53 31.22,32.53 30.22,31.53 30.22,30.43 30.22,29.33 31.22,30.43 31.22,29.33 31.22,31.53 32.32,32.53 32.32,31.53 32.32,30.43 32.32,29.33 33.42,32.53 34.52,32.53 33.42,31.53 34.52,31.53 33.42,30.43 34.52,30.43 33.42,29.33 34.42,29.33 7.65,28.3 8.6,28.93 2.62,27.15 9.97,28.68 10.85,28.68 11.47,28.68 12.22,28.68 12.97,28.68 2.31,35.77 16.12,26.23 13.22,26.78 22.62,28.48 18.97,30.38 19.67,30.53 18.87,29.58 18.52,28.98 18.02,28.43 21.59,27.33 24.62,28.63 27.12,28.4 28.67,28.43 23.32,30.43 23.22,27.18 21.97,31.6 15.62,31.88 15.62,30.98 15.02,30.98 14.42,30.98 11.72,30.68 11.72,29.93 10.18,33.81 11.77,34.86 11.72,29.28 10.42,29.17 10.67,33.15 12.07,33 11.02,33.93 11.37,33.1 10.07,33.15 8.82,33.15 11.27,35.43 7.67,29.02 7.67,29.75 6.95,29.77 2.67,32.58 3.17,33.13 3.87,33.43 4.62,33.53 5.32,33.33 6.02,32.93 6.47,32.43 7.59,33.15 10.27,27.78 8.27,33.15 9.42,33.15 10.27,34.53 9.27,33.78 7.77,35.63 4.88,34.47 15.77,36.33 19.72,34.93 27.5,34.15 6.29,35.63 11.86,36.56 17.32,28.28 23.97,28.68 31.62,36.23 6.07,28.5 4.42,28.51 5.01,25.65 3.46,25.7 1.75,25.7 1.2,27.1 4.01,27.13 7.17,32.43 7.87,32.43 6.71,25.56 10.17,26.83 11.52,27.68 8.47,26.83 16.52,29.68 17.02,26.18 16.57,26.63 12.37,26.68 19.67,28.98 16.67,28.28 15.02,31.88 1.22,28.43 2.55,28.48 4.72,29.43 5.37,29.63 4.02,29.43 3.42,29.68 2.87,30.03 2.57,30.63 2.37,31.28 2.47,31.98 1.22,29.78 1.22,31.52 25.32,28.13 25.9,28 24.72,30.33 25.42,30.33 26.12,30.33 27.32,30.83 24.02,30.33 23.32,28.63 23.27,34.03 22.62,30.53 23.37,31.03 23.62,33.53 23.97,34.03 24.82,34.03 25.52,34.03 26.22,34.03 26.92,34.03 21.97,30.95 18.82,36.13 2.88,34.52 13.27,29.88 13.27,29.23 36.72,25.73 25.42,26.93 25.52,27.53 23.52,26.23 11.07,25.88 6.47,30.58 9.22,28.92 5.92,30.03 7.17,30.58 7.8,30.58 1.45,36.51 1.64,34.4 4.5,35.7 3.67,36.49 8.67,34.63 24.57,27.28 36.12,35.78 34.22,36.28 30.4,36.45 21.97,36.23 20.47,36.18 21.17,36.08 18.27,34.68 14.92,36.56 15.57,34.18 9.12,36.46 20.37,28.68 20.72,26.93 24.22,26.23 24.92,26.23 25.62,26.23 5.47,36.48 10.07,35.73 10.72,36.59 7.42,36.57 7.16,34.51 22.12,34.93 21.37,34.93 20.57,34.93 22.72,31.35 21.27,33.48 17.57,33.98 22.12,28.08 18.97,34.93 19.67,36.13 15.07,35.08 17.52,33.28 20.62,33.2 21.22,32.63 17.52,32.58 19.02,28.23 29.47,36.45 42.52,13.75 43.28,13.75 42.52,12.61 44.04,12.61 43.28,12.61 44.04,13.75 5.45,27.09 6.96,27.09 1.98,39.18 3.26,41.74 7.09,45.57 8.37,41.74 7.09,39.18 12.2,39.18 12.2,45.57 13.48,41.74 17.31,45.57 18.59,41.74 17.31,39.18 21.15,39.18 22.43,45.57 28.82,45.57 40.87,41.24 45.41,41.24 48.39,38.18 48.46,34.09 48.46,29.98 1.98,22.57 7.09,22.57 5.81,20.01 10.92,11.07 5.81,8.51 8.37,14.9 10.92,20.01 13.48,22.57 16.04,20.01 18.59,22.57 23.7,22.57 21.15,20.01 42.87,21.29 32.65,18.74 39.04,17.46 35.21,13.62 22.43,14.9 31.37,9.79 16.04,14.9 28.82,14.9 14.76,5.96 24.98,11.07 18.59,11.07 19.87,5.96 24.98,5.96 30.09,5.96 35.21,5.96 40.32,5.96 40.1,37.53 45.59,26.48 37.76,22.58 48.46,26.43 61.77,28.64 62.03,14.92 57.51,28.38 53.21,27.8 53.27,22.11 57.48,14.84 54.33,18.58
  pour Top (no thermals): 28.62,28.23 36.02,28.23 36.02,33.63 28.62,33.63
  pour VDD-Plane (isolate 0.305, no thermals): 13.82,34.08 13.82,28.93 15.92,28.93 15.92,27.83 24.17,27.83 24.17,35.33 14.52,35.33 14.52,34.08
  pour Top (isolate 0.305, rank 4, no thermals): 0.26,32.24 0.26,47.99 2.8,50.53 2.8,52.56 3.3,53.07 3.81,53.07 67.57,53.07 67.82,53.07 68.33,52.56 68.33,0.74 67.82,0.23 4.07,0.23 2.8,1.5 2.8,12.93 0.26,15.47
  pour GND-Plane (isolate 0.305, no thermals): 0.26,15.47 0.26,48.24 2.8,50.78 2.8,52.56 3.3,53.07 67.82,53.07 68.33,52.56 68.33,0.74 67.82,0.23 4.07,0.23 2.8,1.5 2.8,12.93
  pour Bottom (isolate 0.305, no thermals): 0.26,15.47 0.26,48.24 2.8,50.78 2.8,52.56 3.3,53.07 67.82,53.07 68.33,52.56 68.33,0.74 67.82,0.23 4.07,0.23 2.8,1.5 2.8,12.93
L1
  Top 0.2: LVCO.2 29.7,27.65 30.07,28.03 U1.10
L2
  Top 0.254: U1.11 30.57,27.47 LVCO.1
LED0
  Top 0.254: U1.19 34.57,28.18 34.92,27.83 36.52,27.83 37.82,26.53 | 37.87,26.03 LED1.A 37.87,26.48 37.82,26.53 | 37.82,26.53 37.82,26.58
N$1  (via drill 0.3)
  Top 0.254: X3.1 v22.37,33.93 | U$2.14 v14.77,29.03
  Bottom 0.254: v14.77,29.03 17.22,29.03 arc90 18.27,30.08 18.27,33.33 arc-90 19.17,34.28 22.02,34.28 arc-90 v22.37,33.93
N$2
  Top 0.254: LED1.C R1.4
N$3
  Top 0.254: 10.93,30.62 CH3.1
  Top 0.289: LH2.2 11.47,31.43 arc67 11.92,31.73 arc-67 12.52,32.13 U$2.9
  Top 0.3: CH5.2 10.92,31.43 LH2.2 10.95,30.62 10.93,30.62
  Top 0.406: CH5.2
N$4
  Top 0.3: CH2.1 9.77,31.4 | 9.77,31.4 LH1.2 LH2.1 | 9.77,31.4 9.77,32.23 | 9.77,32.23 CH4.2 | CH5.1 9.77,32.23
  Top 0.406: CH4.2
N$5
  Top 0.254: 8.61,30.64 CH1.1
  Top 0.289: LH1.1 X2.1
  Top 0.3: CH4.1 8.6,32.2 LH1.1 8.61,31.41 8.61,30.64
  Top 0.406: CH4.1
N$6
  Top 0.254: U$2.16 15.77,29.28 15.97,29.08 15.97,27.63 16.27,27.33 R4.4 R5.4
N$7
  Top 0.61: 33.02,47.62 C12.1 33.02,47.59
  Top 0.813: JP2.5 33.02,47.62 | JP5.2 33.02,47.59
  Top 1.016: R15.1 35.52,45.45 JP5.2
N$8
  Top 0.289: U$2.10 12.92,31.63 arc90 12.52,31.23 LPA1.1
N$9
  Top 0.254: LPA2.1 U$2.7
N$10
  Top 0.254: R10.4 24.69,35.57 R11.3 24.96,35.54 25.32,35.18 25.72,35.18 Q2.1
N$11
  Top 0.2: U1.38 30.52,33.33 C9.2
N$12
  Top 0.3: R7.4 19.71,31.79 R9.4 19.85,31.79 CPA10.1 21.03,30.61 CPA8.1 20.51,30.03 LPA4.1
N$14
  Top 0.254: 18.39,31.63 R7.3
  Top 0.289: U$2.3 18.39,31.63
  Top 0.3: R7.3 19.08,32.32 R8.4
N$15
  Top 0.61: R16.1 45.77,18.67 Q3.B
N$17
  Top 0.3: LPA4.2 21.66,30.01 CPA8.2 21.66,29.74 21.87,29.53 | LT3.2 21.87,29.53 | CPA11.1 21.87,29.03 21.87,29.53
N$23
  Top 0.3: LB1.2 23.11,32.24 X3.4 23.17,32.23 23.52,31.88 CB2.1
PB0
  Top 0.254: U1.18 34.07,27.98 34.72,27.33 35.72,27.33 TP12.P$1
PB2/VTCXO  (via drill 0.3)
  Top 0.2: U1.20 36.72,28.53 v36.92,28.33 | v35.12,37.53 27.12,37.53 27.02,37.43 R3.3
  Bottom 0.2: v36.92,28.33 38.32,26.93 43.72,26.93 44.22,27.43 44.22,35.53 43.42,36.33 36.32,36.33 v35.12,37.53
PB3  (via drill 0.3)
  Top 0.254: U1.21 37.07,29.18 37.92,28.33 X1.P9 39.47,28.38 v39.47,28.88 39.67,28.88
  Bottom 0.254: TP14.TP 40.12,28.93 v39.47,28.88
PB4/TX0  (via drill 0.3, 0.5)
  Top 0.254: U1.22 37.67,29.68 38.12,29.48 v41.67,29.48 42.52,29.48 X1.P8
  GND-Plane 0.254: v41.79,24.36 42.42,25 42.42,28.56 41.67,29.31 v41.67,29.48
  Bottom 0.254: 42.37,29.28 TP9.TP 42.12,29.03 v41.67,29.48 | JP3.1 5.08,2.9 11.05,8.87 26.67,8.87 41.79,23.98 v41.79,24.36
PB5/RX0  (via drill 0.3, 0.5)
  Top 0.254: U1.23 39.37,30.18 39.42,30.23 X1.P7 39.67,30.58 v41.57,30.58
  GND-Plane 0.254: v43.06,24.36 43.06,29.1 v41.57,30.58
  Bottom 0.254: v41.57,30.58 42.02,31.03 TP2.TP | JP3.2 7.62,4.55 11.31,8.24 26.93,8.24 v43.06,24.36
PC0
  Top 0.254: U1.17 33.57,27.78 34.72,26.63 35.12,26.63 TP11.P$1
PC1
  Top 0.254: U1.16 33.07,27.48 TP10.P$1
PC2
  Top 0.254: U1.15 32.57,27.18 33.42,26.33 TP7.P$1
PC3
  Top 0.254: U1.14 32.07,26.78 32.22,26.63 TP6.P$1
PC4  (via drill 0.3)
  Top 0.254: U1.13 31.57,26.18 v31.22,25.83 | v11.97,25.78 13.07,25.78 S1.P1
  Bottom 0.254: 31.02,25.63 v31.22,25.83 30.92,25.53 12.22,25.53 v11.97,25.78
RESET_SW
  Top 0.305: IC1.8 44.06,16.22 44.2,16.36 R16.2
RST_N  (via drill 0.3, 0.5)
  Top 0.254: U1.27 36.17,32.18 37.42,33.58 37.82,34.03 v37.95,34.15 38.12,34.33 X1.P3 | R17.2 46.23,22.59 v44.45,24.36
  Top 0.61: Q3.C 46.74,22.56 | 46.74,22.56 R17.2 | 46.74,22.56 46.74,23.83 47.45,24.54 53.12,24.54 C13.2 53.98,25.39 S2.3 S2.1
  GND-Plane 0.254: v44.45,24.36 43.75,25.06 43.75,29.51 42.55,30.71 42.55,32.24 40.63,34.15 v37.95,34.15
  Bottom 0.254: TP4.TP 40.22,33.53 40.07,33.68 38.42,33.68 v37.95,34.15
SCL  (via drill 0.5)
  Top 0.254: IC1.19 41.67,11.34 41.46,11.55 IC1.18 40.71,11.94 v40.62,11.84 | JP4.10 49.78,3.03 46.74,6.08 R13.1 | IC1.23 44.06,10.91 44.35,10.62 45.27,10.62 v45.54,10.9
  Top 0.406: R13.1 46.35,10.9 v45.54,10.9
  Bottom 0.254: v45.54,10.9 41.02,10.9 40.62,11.31 v40.62,11.84
SDA
  Top 0.254: IC1.20 42.56,10.94 42.24,10.62 40.52,10.62 R14.1 40.52,10.58 40.52,8.62 43.18,5.95 46.1,5.95 47.24,4.81 JP4.9
SYSC
  Top 0.254: U1.12 31.07,26.58 30.82,26.33 TP1.P$1
VDDA1
  Top 0.254: U1.1 28.27,32.68 28.12,32.73 C100.2
VDDA2
  Top 0.3: U1.7 28.57,29.68 28.22,29.33 28.22,29.13 C101.1
VSUP  (via drill 0.3, 0.5)
  Top 0.2: U1.36 31.52,33.38 31.52,35.33 v31.57,35.33 31.77,35.43 C105.2
  Top 0.254: v19.47,26.38 18.78,26.38 R5.3 | IC1.21 43.06,10.47 42.97,10.38 C10.1
  Top 0.305: U1.29 35.22,33.33 35.37,33.48 35.37,33.58
  Top 0.406: C103.1 37.02,35.03 C11.1 36.42,34.63 35.37,33.58 | v37.82,35.73 37.77,35.78 | C10.1 v41.8,9.59 v41.79,9.58 | R12.2 45.28,6.9 v45.34,6.84 | R13.2 v49.53,10.52 | R14.2 38.8,9.57 v38.86,9.51
  Top 0.61: R17.1 v49.72,22.59
  Top 0.813: C103.1 37.77,35.78 40.37,35.78 X1.P1
  Top 1.016: R15.2 35.52,42.91 JP5.1
  VDD-Plane 0.406: v41.79,9.58 41.79,9.33 41.76,9.3 | v45.34,6.84 44.83,6.84 | v49.53,10.52 49.53,9.89 | v38.86,9.51 38.86,9.38 38.99,9.25
  VDD-Plane 0.61: v49.72,22.59 50.04,22.59 50.42,22.97
  Bottom 0.406: TP5.TP 39.97,35.03 v39.97,35.73
  other vias: 38.57,35.73 14.02,34.78 39.27,35.73 40.57,35.73 13.57,35.18 15.4,28.38 14.22,28.4 14.82,28.25 13.12,34.78 32.39,41 33.66,41 34.86,41
  pour Top (isolate 0.1, no thermals): 13.02,33.78 13.97,33.78 13.97,34.38 14.27,34.58 14.27,35.43 12.92,35.43 12.92,34.58 13.02,34.43
  pour Top (isolate 0.17, rank 2, no thermals): 14.07,30.13 14.07,27.48 15.62,27.48 15.62,30.13
  pour Top (isolate 0.305, rank 2, no thermals): 31.69,43.03 31.69,40.68 32.39,39.99 34.86,39.99 35.44,40.56 35.44,43.1 35.37,43.16 31.82,43.16
  pour VDD-Plane (isolate 0.254, rank 2, no thermals): 0.26,15.47 0.26,48.24 2.8,50.78 2.8,52.56 3.3,53.07 67.82,53.07 68.33,52.56 68.33,0.74 67.82,0.23 4.07,0.23 2.8,1.5 2.8,12.93
VTCXO
  Top 0.254: C102.2 Q2.4 25.57,36.33 25.57,37.23 25.77,37.43 R3.4

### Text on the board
tNames: ON | ON Semiconductor | US Sigfox | Connector position | Reset SW | IC1
bNames: (c) AXSEM AG, 2015 / F143-MINI-KIT-SMA-22dB / v 1.0
Document: Coplanar Wave Guide with GND Plane / Spacing 0.25mm, Prepreg thickness 0.156mm / -> 0.289mm Trace Width @ 50Ohm
bDocu: (C) AXSEM AG, 2017 | REV 1-0-2 | F143-MINI-DVK-FE-SMA | 902 MHz / 48 MHz TCXO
